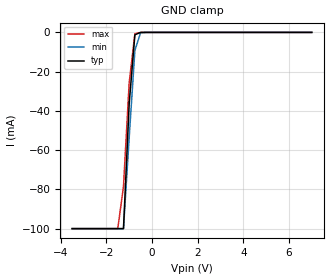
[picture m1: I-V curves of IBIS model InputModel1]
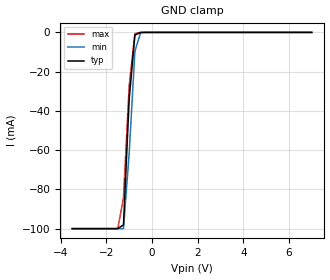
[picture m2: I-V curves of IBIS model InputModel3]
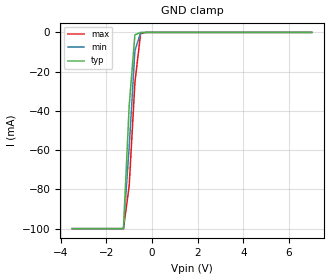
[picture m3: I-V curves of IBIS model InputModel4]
[IBIS Ver]   2.1
[File name]   e_016xs3.ibs   | e_= TSOP, f016xs= abbr chip name, 3= 3.3V Vcc
[File Rev]   2.40
[Date]   05-February-1996
[Source]   File generated from lab measurements at Intel Corporation
[Notes]   Rev 2.00 fixes simulation model flaw.
   Rev 2.01 fixes typo errors in comments only.
   Rev 2.10 implements improvements for Quad parser IBIS2XTK:
   * adds zero current [POWER_clamp] to input models
   * changes model name from "I/O" to "InputOutput"
   * changes model type "Open_Drain" to "Open_drain"
   Rev 2.20 adds required dV/dt_r for OpenDrainOutput.
   Rev 2.30 adds 3/5# pin to pin #1.  The input model remains
   the same as it was included in rev 2.20, though the pin
   was a no connect in that model.
   Rev 2.40 All data was replaced by actual measurements
   performed in a lab.
[Disclaimer] INTEL DEVELOPER'S SOFTWARE LICENSE AGREEMENT
| BY USING THIS SOFTWARE, YOU ARE AGREEING TO BE BOUND
| BY THE TERMS OFTHIS AGREEMENT.  DO NOT USE THE SOFTWARE
| UNTIL YOU HAVE CAREFULLY READAND AGREED TO THE FOLLOWING
| TERMS AND CONDITIONS.  IF YOU DO NOT AGREETO THE TERMS
| OF THIS AGREEMENT, PROMPTLY RETURN THE SOFTWARE PACKAGE
| ANDANY ACCOMPANYING ITEMS.
| IF YOU USE THIS SOFTWARE, YOU WILL BE BOUND BY THE TERMS
| OF THIS AGREEMENT
| LICENSE: Intel Corporation ("Intel") grants you the non-exclusive right
| to use the enclosed software program ("Software").  You will not use,
| copy, modify, rent, sell or transfer the Software or any portion
| thereof, except as provided in this Agreement.
| System OEM Developers may:
| 1.   Copy the Software for support, backup or archival purposes;
| 2.   Install, use, or distribute Intel owned Software in object code
|   only;
| 3.   Modify and/or use Software source code that Intel directly makes
|   available to you as an OEM Developer;
| 4.   Install, use, modify, distribute, and/or make or have made
|   derivatives ("Derivatives") of Intel owned Software under the
|   terms and conditions in this Agreement, ONLY if you are a System
|   OEM Developer and NOT an end-user.
| RESTRICTIONS:
| YOU WILL NOT:
| 1.   Copy the Software, in whole or in part, except as provided for
|   in this Agreement;
| 2.   Decompile or reverse engineer any Software provided in object
|   code format;
| 3.   Distribute any Software or Derivative code to any end-users,
|   unless approved by Intel in a prior writing.
| TRANSFER: You may transfer the Software to another OEM
| Developer if thereceiving party agrees to the terms of this
| Agreement at the sole risk of any receiving party.
| OWNERSHIP AND COPYRIGHT OF SOFTWARE:
| Title to the Software and all copies thereof remain with Intel
| or its vendors.  The Software iscopyrighted and is protected by
| United States and international copyright laws.  You will not
| remove the copyright notice from the Software.  You agree to
| prevent any unauthorized copying of the Software.
| DERIVATIVE WORK: OEM Developers that make or have made
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[Copyright]   Copyright 1994,1996, Intel Corporation, All Rights Reserved
[Component]   E28F016XS   | 56-lead TSOP package, 28F016XS
[Manufacturer]  Intel   | Synchronous Flash Memory
|   | operating in 3.3V Vcc range
[Package]
| Variable   typ   min   max
|The following values apply for the Copper leadframe.
R_pkg   48m   41m   54m
L_pkg   4.92nH   4.44nH   5.39nH
C_pkg   0.48pF   0.45pF   0.50pF
|The following values apply for the Alloy-42 leadframe.
|R_pkg   195m   180m   210m
|L_pkg   4.92nH   4.44nH   5.39nH
|C_pkg   0.48pF   0.45pF   0.50pF
|********************Pin Definitions*************************************
[Pin]   signal_name   model_name   R_pin   L_pin   C_pin
  1   3/5#   InputModel1
  2   CE1#   InputModel1
  3   NC   InputModel2
  4   A20   InputModel3
  5   A19   InputModel3
  6   A18   InputModel1
  7   A17   InputModel1
  8   A16   InputModel1
  9   VCC   POWER
 10   A15   InputModel1
 11   A14   InputModel3
 12   A13   InputModel1
 13   A12   InputModel1
 14   CE0#   InputModel1
 15   VPP   POWER
 16   RP#   InputModel4
 17   A11   InputModel1
 18   A10   InputModel1
 19   A9   InputModel1
 20   A8   InputModel1
 21   GND   GND
 22   A7   InputModel1
 23   A6   InputModel1
 24   A5   InputModel1
 25   A4   InputModel1
 26   A3   InputModel1
 27   A2   InputModel1
 28   A1   InputModel1
 29   CLK   InputModel5
 30   ADV#   InputModel5
 31   BYTE#   InputModel1
 32   A0   InputModel1
 33   DQ0   InputOutput
 34   DQ8   InputOutput
 35   DQ1   InputOutput
 36   DQ9   InputOutput
 37   VCC   POWER
 38   DQ2   InputOutput
 39   DQ10   InputOutput
 40   DQ3   InputOutput
 41   DQ11   InputOutput
 42   GND   GND
 43   VCC   POWER
 44   DQ4   InputOutput
 45   DQ12   InputOutput
 46   DQ5   InputOutput
 47   DQ13   InputOutput
 48   GND   GND
 49   DQ6   InputOutput
 50   DQ14   InputOutput
 51   DQ7   InputOutput
 52   DQ15   InputOutput
 53   RY/BY#   OpenDrainOutput
 54   OE#   InputModel1
 55   WE#   InputModel4
 56   WP#   InputModel1
|********************Input Model 2*****************************************
[Model]   InputModel2
Model_type   Input
|   for pin3(NC)
Vinl = 0.8V
Vinh = 2.0V
| Variable   typ   min   max
C_comp   5.61p   NA   7.6p
[Voltage Range]   3.3V   3.0V   3.6V
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| Models and submodels in the file (7): InputModel1 (Input), InputModel2 (Input), InputModel3 (Input), InputModel4 (Input), InputModel5 (Input), InputOutput (I/O), OpenDrainOutput (Open_drain)
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|*********************Inoput Model 1***************************************
[Model]   InputModel1
Model_type   Input
|   for pin1(3/5#), CE1#, CE0#, OE#, WP#, BYTE#, A[18:15], A[13:0]
Vinl = 0.8V
Vinh = 2.0V
| Variable   typ   min   max
C_comp   5.61p   NA   7.6p
[Voltage Range]   3.3V   3.0V   3.6V
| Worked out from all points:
|   GND clamp passes 1 mA (typ) near -0.71 V on its own axis
[GND_clamp]
|Voltage I(typ)   I(min)   I(max)
-3.5V     -99.93mA   -99.94mA   -99.95mA
-1.5V     -99.93mA   -99.94mA   -99.95mA
-1.25V    -99.93mA   -99.94mA   -78.52mA
-1V       -36.25mA   -53.59mA   -25.61mA
-750mV    -1.199mA   -9.118mA   -666.9uA
-500mV    -23uA      -169.3uA   -33.07uA
7V        0A         0A         0A
[POWER_clamp]
| Input buffer circuits of this product do not intrinsically
| require a [POWER_clamp] definition.  This zero current
| [POWER_clamp] is provided for compatibility with some ibis
| parsers.
|   Voltage  I(typ)   I(min)   I(max)
-3.3V     0A         0A         0A
-3V       0A         0A         0A
6.3V      0A         0A         0A
6.6V      0A         0A         0A
|*******************Input Model 3**************************************
[Model]   InputModel3
Model_type   Input
|   for A[20], A[19], A[14]
Vinl = 0.8V
Vinh = 2.0V
| Variable   typ   min   max
C_comp   5.61p   NA   7.6p
[Voltage Range]   3.3V   3.0V   3.6V
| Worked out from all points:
|   GND clamp passes 1 mA (typ) near -0.68 V on its own axis
[GND_clamp]
|Voltage I(typ)   I(min)   I(max)
-3.5V     -99.93mA   -99.94mA   -99.95mA
-1.5V     -99.93mA   -99.94mA   -99.95mA
-1.25V    -98.01mA   -99.94mA   -84.37mA
-1V       -33.88mA   -61.45mA   -27.19mA
-750mV    -1.338mA   -9.608mA   -639.5uA
-500mV    -54.63uA   -152.9uA   0A
7V        0A         0A         0A
[POWER_clamp]
| Input buffer circuits of this product do not intrinsically
| require a [POWER_clamp] definition.  This zero current
| [POWER_clamp] is provided for compatibility with some ibis
| parsers.
|   Voltage  I(typ)   I(min)   I(max)
-3.3V     0A         0A         0A
-3V       0A         0A         0A
6.3V      0A         0A         0A
6.6V      0A         0A         0A
|*********************Input Model 4*************************************
[Model]   InputModel4
Model_type   Input
|   for RP#, WE#
Vinl = 0.8V
Vinh = 2.0V
| Variable   typ   min   max
C_comp   5.61p   NA   7.6p
[Voltage Range]   3.3V   3.0V   3.6V
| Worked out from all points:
|   GND clamp passes 1 mA (typ) near -0.70 V on its own axis
[GND_clamp]
|Voltage I(typ)   I(min)   I(max)
-3.5V     -99.94mA   -99.94mA   -99.95mA
-1.25V    -99.94mA   -99.94mA   -99.95mA
-1V       -37.36mA   -58.41mA   -78.12mA
-750mV    -1.233mA   -9.326mA   -25.63mA
-500mV    -23.22uA   -151.2uA   -617uA
-250mV    0A         0A         0A
7V        0A         0A         0A
[POWER_clamp]
| Input buffer circuits of this product do not intrinsically
| require a [POWER_clamp] definition.  This zero current
| [POWER_clamp] is provided for compatibility with some ibis
| parsers.
|   Voltage  I(typ)   I(min)   I(max)
-3.3V     0A         0A         0A
-3V       0A         0A         0A
6.3V      0A         0A         0A
6.6V      0A         0A         0A
